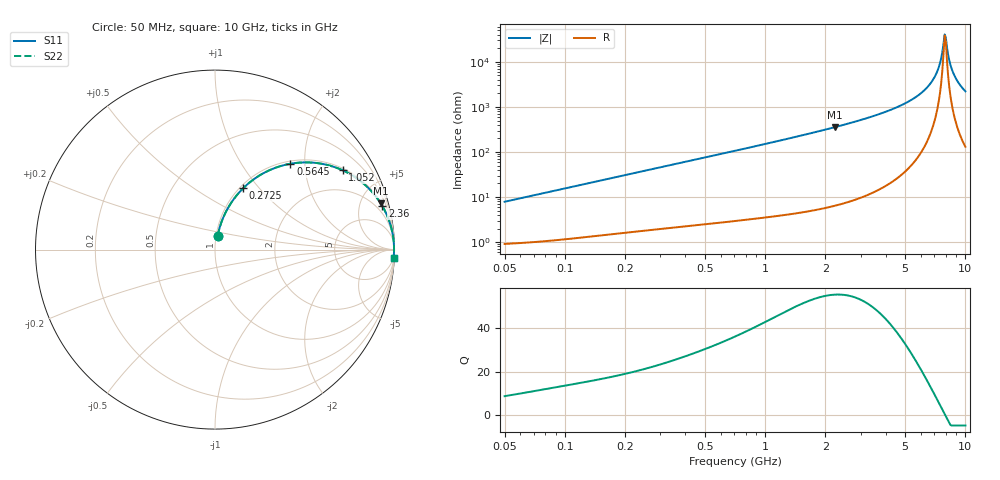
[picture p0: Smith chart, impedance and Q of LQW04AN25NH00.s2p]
!Murata Part Number: LQW04AN25NH00
!These Parameters are Measured in Series Mode Connection
!  o--[Z]--o
!Port1  Port2
!  o-------o
!Freq. Start=50[MHz] Stop=10[GHz], 401[Steps]
# Hz S RI R 50
!Freq.(Hz)	S 11(Real)	S 11(Imag)	S 21(Real)	S 21(Imag)	S 12(Real)	S 12(Imag)	S 22(Real)	S 22(Imag)
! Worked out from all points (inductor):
!   401 points, 50 MHz to 10 GHz, reference 50 ohm
!   read as one part in series: L = 24.8 nH near 51.34 MHz
!   highest Q = 55.6 at 2.239 GHz (marker M1), where L = 25.4 nH
!   self-resonance near 7.879 GHz
!   S11 on the Smith chart (normalised r, x): 50 MHz: 1.02, +0.16; 272.5 MHz: 1.04, +0.82; 564.5 MHz: 1.05, +1.69; 1.052 GHz: 1.07, +3.17; 2.36 GHz: 1.14, +7.61; 10 GHz: 4, -44
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5e7  0.0149 0.0761  0.9851 -0.0761  0.9851 -0.0761  0.0149 0.0761
1.214486e8  0.045 0.1763  0.955 -0.1763  0.955 -0.1763  0.045 0.1763
2.72458e8  0.1563 0.3413  0.8437 -0.3413  0.8437 -0.3413  0.1563 0.3413
2.949953e8  0.1763 0.36  0.8237 -0.36  0.8237 -0.36  0.1763 0.36
5.645355e8  0.4201 0.4783  0.5799 -0.4783  0.5799 -0.4783  0.4201 0.4783
7.071068e8  0.5286 0.4856  0.4714 -0.4856  0.4714 -0.4856  0.5286 0.4856
1.052113e9  0.7112 0.442  0.2888 -0.442  0.2888 -0.442  0.7112 0.442
1.717543e9  0.8713 0.3256  0.1287 -0.3256  0.1287 -0.3256  0.8713 0.3256
2.23851e9  0.9235 0.2569  0.0765 -0.2569  0.0765 -0.2569  0.9235 0.2569
2.360312e9  0.9316 0.2436  0.0684 -0.2436  0.0684 -0.2436  0.9316 0.2436
4.171863e9  0.9834 0.1167  0.0166 -0.1167  0.0166 -0.1167  0.9834 0.1167
5.509778e9  0.9934 0.0644  0.00661 -0.0644  0.00661 -0.0644  0.9934 0.0644
6.54512e9  0.9965 0.0337  0.00347 -0.0337  0.00347 -0.0337  0.9965 0.0337
7.276762e9  0.9975 0.015  0.00254 -0.015  0.00254 -0.015  0.9975 0.015
7.472112e9  0.9976 0.0103  0.00242 -0.0103  0.00242 -0.0103  0.9976 0.0103
7.775012e9  0.9977 0.00314  0.00233 -0.00314  0.00233 -0.00314  0.9977 0.00314
7.878683e9  0.9977 0.000762  0.00233 -0.000762  0.00233 -0.000762  0.9977 0.000762
8.090191e9  0.9976 -0.00403  0.00236 0.00403  0.00236 0.00403  0.9976 -0.00403
8.418147e9  0.9975 -0.0113  0.00249 0.0113  0.00249 0.0113  0.9975 -0.0113
8.759398e9  0.9972 -0.0187  0.00275 0.0187  0.00275 0.0187  0.9972 -0.0187
9.359165e9  0.9965 -0.0313  0.00347 0.0313  0.00347 0.0313  0.9965 -0.0313
1e10  0.9954 -0.0445  0.00462 0.0445  0.00462 0.0445  0.9954 -0.0445
